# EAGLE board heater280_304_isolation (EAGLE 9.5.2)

Size 173.6 x 210 mm. Coordinates in mm from the lower left corner, seen from the top.
Outline: 0,0 0,210 71.8,210 71.8,200 101.8,200 101.8,210 173.6,210 173.6,0 0,0
Copper layers (1*16): Top 0.035mm / dielectric 1.5mm / Bottom 0.035mm
Design rules "default": minimum track width 6mil, minimum drill 0.35mm, track to track 6mil, track to pad 6mil, pad to pad 6mil, via to via 6mil, smd to smd 6mil, copper to edge 40mil, drill to drill 6mil, minimum pad ring 10mil, minimum via ring 8mil, stop-mask expansion 4mil, vias tented up to drill 0mil, thermal gap 10mil

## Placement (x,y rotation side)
U$1  [CE-4MM]  0.84,194.13 0 top

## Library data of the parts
U$1 = logo

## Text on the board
tPlace: ECS, Am Wenigerflur 14, 54498 Piesport | HEATER280_304 | ISOLATION PLATE / (END PLATE)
